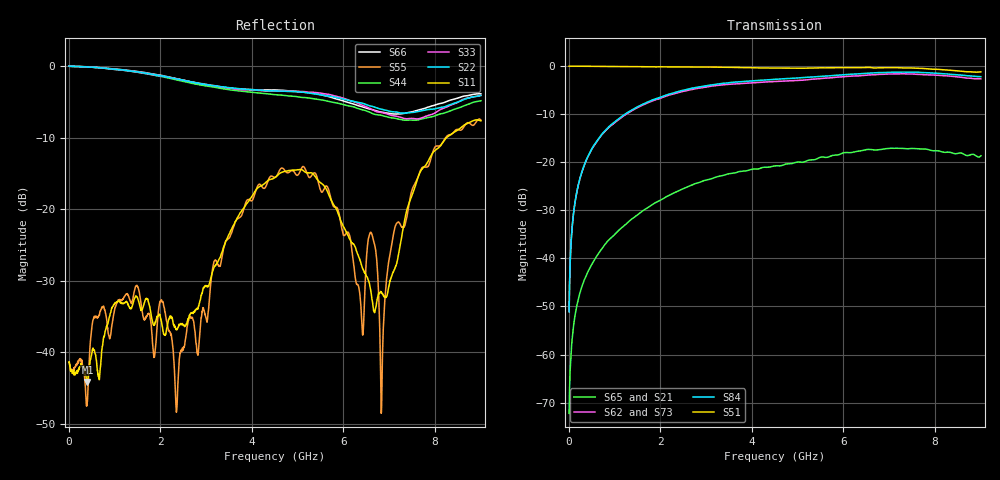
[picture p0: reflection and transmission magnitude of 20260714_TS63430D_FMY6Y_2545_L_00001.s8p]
# GHz S DB R 50
! CMT, SN0916, 25263762, 26.7.0
! Date: 15.07.2026 14:51:57
! Data: Format
! Freq S1.1:dB/Ang S1.2:dB/Ang S1.3:dB/Ang S1.4:dB/Ang S1.5:dB/Ang S1.6:dB/Ang S1.7:dB/Ang S1.8:dB/Ang
!  S2.1:dB/Ang S2.2:dB/Ang S2.3:dB/Ang S2.4:dB/Ang S2.5:dB/Ang S2.6:dB/Ang S2.7:dB/Ang S2.8:dB/Ang
!  S3.1:dB/Ang S3.2:dB/Ang S3.3:dB/Ang S3.4:dB/Ang S3.5:dB/Ang S3.6:dB/Ang S3.7:dB/Ang S3.8:dB/Ang
!  S4.1:dB/Ang S4.2:dB/Ang S4.3:dB/Ang S4.4:dB/Ang S4.5:dB/Ang S4.6:dB/Ang S4.7:dB/Ang S4.8:dB/Ang
!  S5.1:dB/Ang S5.2:dB/Ang S5.3:dB/Ang S5.4:dB/Ang S5.5:dB/Ang S5.6:dB/Ang S5.7:dB/Ang S5.8:dB/Ang
!  S6.1:dB/Ang S6.2:dB/Ang S6.3:dB/Ang S6.4:dB/Ang S6.5:dB/Ang S6.6:dB/Ang S6.7:dB/Ang S6.8:dB/Ang
!  S7.1:dB/Ang S7.2:dB/Ang S7.3:dB/Ang S7.4:dB/Ang S7.5:dB/Ang S7.6:dB/Ang S7.7:dB/Ang S7.8:dB/Ang
!  S8.1:dB/Ang S8.2:dB/Ang S8.3:dB/Ang S8.4:dB/Ang S8.5:dB/Ang S8.6:dB/Ang S8.7:dB/Ang S8.8:dB/Ang
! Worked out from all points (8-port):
!   2001 points, 10 MHz to 9 GHz, reference 50 ohm
!   strongest paths, dB at 10 MHz, 2.257 GHz, 4.505 GHz, 6.753 GHz, 9 GHz:
!     S51: -0.1, -0.2, -0.5, -0.4, -1.3
!     S84: -51.1, -5.7, -2.8, -1.4, -2.3
!     S62: -51.0, -5.9, -3.3, -1.8, -2.7
!     S73: -51.3, -6.1, -3.3, -1.7, -2.7
!     S65: -72.2, -26.6, -20.8, -17.5, -18.7
!     S21: -72.2, -26.7, -20.8, -17.3, -18.7
!   lowest |S11| = -44.1 dB at 410.1 MHz (marker M1), VSWR 1.01, Z = 50.3 - j0.568 ohm
!   |S11| at or under -10 dB: start of sweep to 8.249 GHz
